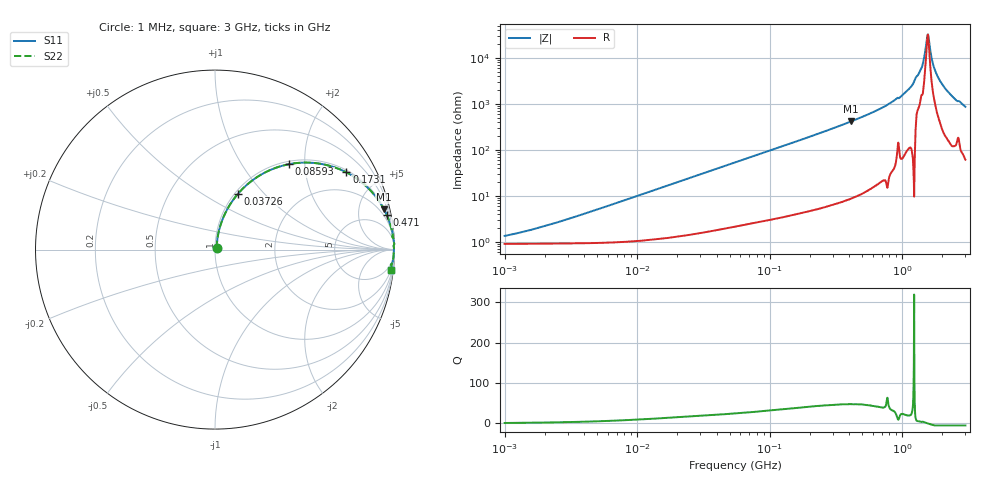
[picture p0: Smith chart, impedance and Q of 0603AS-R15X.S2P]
!s-Parameter Generated by FASTRON Sdn. Bhd.
!FASTRON P/N : 0603AS-R15X
!Keysight Technologies: E4991B_MY54100416_A.01.15
!Date created: Wed Sep 27 15:49:48 2023
!Version  : Rev01 Wed Sep 27 15:49:48 2023
!Data & Calibration Information:
!Freq	S11	S21	S12	S22
!PortZ  Port1:50+j0  Port2:50+j0
!When reading reference impedance value at option line is always used.
! Remarks : This data is being provided solely for informational purposes.
# Hz S dB R 50
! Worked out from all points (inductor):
!   1601 points, 1 MHz to 3 GHz, reference 50 ohm
!   read as one part in series: L = 160 nH near 2.775 MHz
!   highest Q = 47.6 at 411.5 MHz (marker M1), where L = 162 nH
!   self-resonance near 1.558 GHz
!   S11 on the Smith chart (normalised r, x): 1 MHz: 1.02, +0.02; 37.26 MHz: 1.03, +0.73; 85.93 MHz: 1.06, +1.66; 173.1 MHz: 1.09, +3.35; 471 MHz: 1.21, +9.78; 3 GHz: 2, -17
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1000000  -37.42 47.4  -0.08 -0.6  -0.08 -0.6  -37.42 47.4
3804036  -28.20 74.0  -0.09 -2.2  -0.09 -2.2  -28.20 74.0
1.447069e7  -17.01 77.3  -0.19 -8.1  -0.19 -8.1  -17.01 77.3
3.72584e7  -9.42 67.5  -0.68 -19.7  -0.68 -19.7  -9.42 67.5
5.477226e7  -6.69 60.1  -1.23 -27.6  -1.23 -27.6  -6.69 60.1
8.593077e7  -4.02 49.1  -2.42 -39.0  -2.42 -39.0  -4.02 49.1
1.731398e8  -1.42 30.5  -5.90 -58.1  -5.90 -58.1  -1.42 30.5
2.083556e8  -1.03 26.0  -7.15 -62.6  -7.15 -62.6  -1.03 26.0
4.114912e8  -0.28 13.4  -12.70 -75.4  -12.70 -75.4  -0.28 13.4
4.710174e8  -0.21 11.5  -14.00 -77.3  -14.00 -77.3  -0.21 11.5
7.925923e8  -0.06 5.6  -20.14 -83.0  -20.14 -83.0  -0.06 5.6
9.779672e8  -0.05 3.9  -23.33 -83.6  -23.33 -83.6  -0.05 3.9
1.188719e9  -0.02 2.2  -28.16 -85.8  -28.16 -85.8  -0.02 2.2
1.388188e9  -0.04 0.9  -35.39 -74.5  -35.39 -74.5  -0.04 0.9
1.444887e9  -0.03 0.7  -38.57 -75.0  -38.57 -75.0  -0.03 0.7
1.526649e9  -0.03 0.2  -47.02 -47.3  -47.02 -47.3  -0.03 0.2
1.565327e9  -0.03 -0.0  -50.27 5.5  -50.27 5.5  -0.03 -0.0
1.604986e9  -0.03 -0.2  -46.26 51.3  -46.26 51.3  -0.03 -0.2
1.738771e9  -0.03 -0.9  -35.93 76.9  -35.93 76.9  -0.03 -0.9
1.921792e9  -0.04 -1.7  -30.29 81.1  -30.29 81.1  -0.04 -1.7
2.41921e9  -0.07 -4.0  -23.08 81.1  -23.08 81.1  -0.07 -4.0
3e9  -0.13 -6.5  -18.92 79.5  -18.92 79.5  -0.13 -6.5
